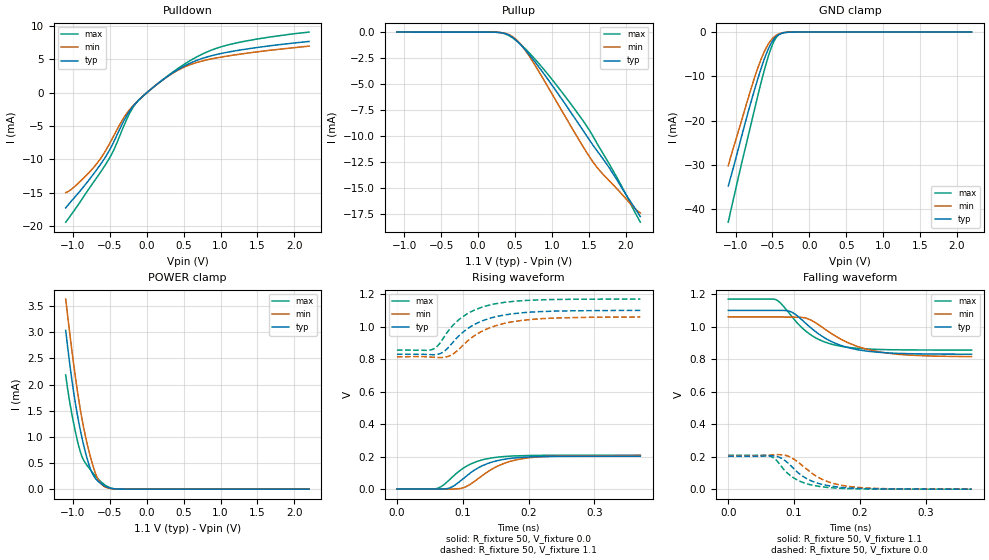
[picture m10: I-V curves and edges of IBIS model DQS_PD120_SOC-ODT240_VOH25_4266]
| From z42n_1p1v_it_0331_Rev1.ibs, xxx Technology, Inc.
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| DQS_PD120_SOC-ODT240_VOH25_4266
| (120 Ohm Pulldown, 240 Ohm System ODT Setting, VOH=VDDQ/2.5, 3200-4266Mbps)
[Model]   DQS_PD120_SOC-ODT240_VOH25_4266
Model_type   I/O
Vinl = 160.000mV
Vinh = 280.000mV
Vmeas = 220.000mV
Vref = 0.0mV
Cref = 0.0pF
Rref = 240.000Ohm
|   typ   min   max
|C_comp   0.849pF   0.799pF   0.899pF
C_comp_pullup   0.4245pF   0.3995pF   0.4495pF
C_comp_pulldown   0.4245pF   0.3995pF   0.4495pF
| Note: C_comp changes when the ODT circuit is enabled.
[Model Spec]
| Input threshold voltage corners
Vinl   0.1600V   0.1520V   0.1740V
Vinh   0.2800V   0.2720V   0.2940V
| Measurement voltage corners
Vmeas   0.2200V   0.2120V   0.2340V
| Timing spec test load voltage corners
Vref   0.0000V   0.0000V   0.0000V
| Dynamic Overshoot Parameters from LPDDR4 Specification
D_overshoot_ampl_h   0.30   NA   NA
D_overshoot_ampl_l   0.30   NA   NA
D_overshoot_area_h   0.1n   NA   NA
D_overshoot_area_l   0.1n   NA   NA
[Voltage Range]   1.1000V   1.0600V   1.1700V
[Pullup Reference]   1.1000V   1.0600V   1.1700V
| Junction Temperature (Ambient temp is 35C typ 95C min -40C max)
[Temperature Range]   50.0   110.0   -40.0
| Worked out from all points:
|   slope of the pulldown table from 0 to 0.165 V, typ, clamps not added: 110 ohm
|   slope of the pullup table from 0 to 0.165 V, typ, clamps not added: 52.6 kohm
|   GND clamp passes 1 mA (typ) near -0.45 V on its own axis
|   POWER clamp passes 1 mA (typ) near -0.88 V on its own axis
|   rising waveform, R_fixture 50, V_fixture 0.0: 20-80 % time 47.7ps typ, 51.9ps min, 43.9ps max; typ from 0 V to 0.203 V
|   falling waveform, R_fixture 50, V_fixture 1.1: 20-80 % time 60.6ps typ, 70.1ps min, 51.4ps max; typ from 1.1 V to 0.831 V
|   rising waveform, R_fixture 50, V_fixture 1.1: 20-80 % time 56.1ps typ, 59.1ps min, 51.7ps max; typ from 0.83 V to 1.1 V
|   falling waveform, R_fixture 50, V_fixture 0.0: 20-80 % time 42.6ps typ, 48.4ps min, 37.8ps max; typ from 0.203 V to 0 V
[Pulldown]
|   Voltage   I(typ)   I(min)   I(max)
-1.1V     -17.26mA   -14.96mA   -19.4mA
-918.5mV  -14.9mA    -13.45mA   -16.6mA
-674.3mV  -11.46mA   -10.57mA   -12.65mA
-469.7mV  -7.838mA   -6.913mA   -9.064mA
-298.1mV  -3.934mA   -3.521mA   -4.632mA
-176mV    -1.9mA     -1.832mA   -2.026mA
-57.2mV   -573uA     -567.7uA   -564.7uA
223.3mV   1.982mA    1.959mA    2.006mA
559.9mV   4.272mA    4.07mA     4.612mA
979mV     5.796mA    5.269mA    6.765mA
1.458V    6.701mA    6.056mA    7.958mA
2.2V      7.669mA    6.972mA    9.07mA
[GND Clamp]
|   Voltage   I(typ)   I(min)   I(max)
-1.1V     -34.75mA   -30.2mA    -42.92mA
-941.6mV  -25.02mA   -21.25mA   -31.33mA
-786.5mV  -15.53mA   -12.6mA    -20.5mA
-723.8mV  -11.94mA   -9.346mA   -16.11mA
-664.4mV  -8.74mA    -6.576mA   -12.08mA
-588.5mV  -5.114mA   -3.68mA    -7.305mA
-519.2mV  -2.565mA   -1.833mA   -3.663mA
-466.4mV  -1.294mA   -941.8uA   -1.691mA
-413.6mV  -563.1uA   -417.1uA   -621.1uA
-350.9mV  -166.1uA   -126.6uA   -147.6uA
-238.7mV  -9.056uA   -8.494uA   -5.049uA
2.2V      0A         0A         0A
[Pullup]
|   Voltage   I(typ)   I(min)   I(max)
-1.1V     1.369uA    2.477uA    453.9nA
262.9mV   -21.59uA   -21.11uA   -22.16uA
385mV     -183.8uA   -152.5uA   -220.4uA
503.8mV   -707uA     -636.9uA   -738.7uA
609.4mV   -1.453mA   -1.458mA   -1.392mA
738.1mV   -2.555mA   -2.79mA    -2.331mA
1.022V    -5.289mA   -6.172mA   -4.721mA
1.448V    -9.706mA   -11.28mA   -8.764mA
1.642V    -11.68mA   -13.25mA   -11.05mA
1.89V     -14.28mA   -15.11mA   -14.06mA
2.114V    -16.79mA   -16.85mA   -17.14mA
2.2V      -17.73mA   -17.38mA   -18.26mA
[POWER Clamp]
|   Voltage   I(typ)   I(min)   I(max)
-1.1V     3.033mA    3.633mA    2.184mA
-1.054V   2.491mA    3.082mA    1.736mA
-981.2mV  1.753mA    2.275mA    1.183mA
-911.9mV  1.201mA    1.61mA     764.6uA
-855.8mV  837.7uA    1.171mA    552.1uA
-779.9mV  447.8uA    701.5uA    396.3uA
-707.3mV  225.4uA    345.4uA    267.6uA
-651.2mV  138.6uA    162.3uA    181.2uA
-595.1mV  80.75uA    68.29uA    109.2uA
-486.2mV  16.69uA    10.22uA    20.94uA
-367.4mV  1.19uA     878nA      944.5nA
2.2V      0A         0A         0A
[Ramp]
|   typ   min   max
| 20% - 80%
dV/dt_r   121.46m/47.69p   123.76m/51.89p   125.27m/43.89p
dV/dt_f   161.60m/60.65p   146.48m/70.12p   188.39m/51.38p
| 25% - 75%
|dV/dt_r   101.22m/37.88p   103.13m/41.35p   104.39m/34.83p
|dV/dt_f   134.67m/48.16p   122.07m/55.68p   156.99m/40.75p
R_load = 50
[Rising Waveform]
R_fixture = 50
V_fixture = 0.0
|   Time   V(typ)   V(min)   V(max)
0s        321.6uV    257.2uV    238.4uV
59ps      232uV      159.8uV    2.748mV
78ps      4.922mV    205.4uV    51mV
88ps      24.46mV    1.227mV    88.72mV
105ps     79.63mV    15.23mV    139.6mV
125ps     134.4mV    69.62mV    174.9mV
149ps     171.9mV    133.5mV    195.1mV
177ps     191.3mV    176.2mV    204.3mV
211ps     199.5mV    197.3mV    207.7mV
370ps     202.8mV    206.5mV    209mV
[Falling Waveform]
R_fixture   = 50
V_fixture   = 1.1
V_fixture_min = 1.06
V_fixture_max = 1.17
|   Time   V(typ)   V(min)   V(max)
0s        1.1V       1.06V      1.17V
72ps      1.1V       1.06V      1.167V
80ps      1.1V       1.06V      1.144V
96ps      1.091V     1.059V     1.065V
121ps     1.009V     1.049V     963mV
144ps     937.9mV    993.4mV    910.1mV
165ps     894.3mV    937.7mV    884.4mV
197ps     858.2mV    877.8mV    866.6mV
238ps     839.7mV    839.7mV    858.9mV
370ps     830.7mV    815.9mV    856mV
[Rising Waveform]
R_fixture   = 50
V_fixture   = 1.1
V_fixture_min = 1.06
V_fixture_max = 1.17
|   Time   V(typ)   V(min)   V(max)
0s        830.4mV    814.6mV    855.9mV
56ps      827.3mV    811.8mV    863.6mV
72ps      848.8mV    811.3mV    938.7mV
83ps      894mV      826.4mV    998.6mV
95ps      947.2mV    864.4mV    1.046V
119ps     1.016V     948mV      1.104V
148ps     1.059V     1.003V     1.14V
178ps     1.08V      1.032V     1.156V
222ps     1.093V     1.05V      1.166V
370ps     1.1V       1.06V      1.17V
[Falling Waveform]
R_fixture = 50
V_fixture = 0.0
|   Time   V(typ)   V(min)   V(max)
0s        202.9mV    206.6mV    209.1mV
58ps      204.9mV    207.9mV    208.6mV
75ps      200.4mV    212.7mV    170.2mV
89ps      167.9mV    206.3mV    102.9mV
101ps     120.6mV    181.7mV    65.92mV
118ps     68.22mV    127.5mV    35.55mV
138ps     34.79mV    70.77mV    17.25mV
164ps     14.65mV    31.21mV    6.844mV
201ps     4.477mV    9.917mV    2.032mV
370ps     413.3uV    419.9uV    267uV
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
